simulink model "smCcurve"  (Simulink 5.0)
settings: Solver=ode45  StartTime=0.0  StopTime=0  MaxStep=1  RelTol=1e-6
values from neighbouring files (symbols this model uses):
  Ef = parEf(m)    [Ccurverun.m]
  Ra = .95    (= 0.95)    [altwdgs.m]    (also in Ccurverun.m = 0.018)
  Vs = abs(Vas)    [calc0.m]    (also in Ccurverun.m = 1; IMabc2.m = 1; IMabcrun0.m = Vll*sqrt(2/3); IMabcrun1.m = Vll*sqrt(2/3))
  Xd = 1.15    [Ccurverun.m]
  Xq = 0.75    [Ccurverun.m]
undefined symbols (not defined in the file or in its folder): phi
libraries: simulink x2

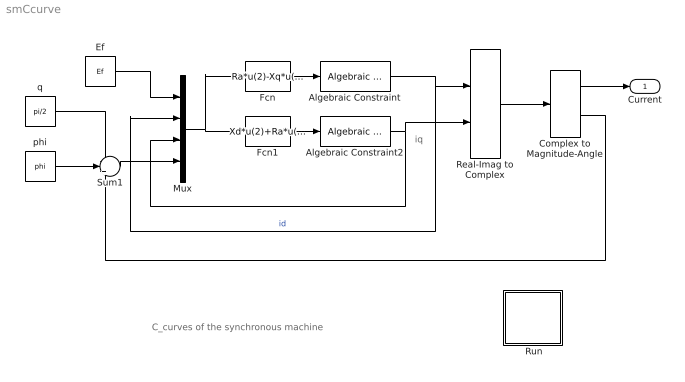
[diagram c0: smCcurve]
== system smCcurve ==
  note: iq
  note: C_curves of the synchronous machine
  " Run" : Subsystem
  Algebraic Constraint : simulink/Math Operations/Algebraic Constraint  z0=.1
  Algebraic Constraint2 : simulink/Math Operations/Algebraic Constraint  z0=0.3
  Complex to Magnitude-Angle : ComplexToMagnitudeAngle
  Ef : Constant  Value=Ef
  Fcn : Fcn  Expr=Ra*u(2)-Xq*u(3)+Vs*sin(u(4))
  Fcn1 : Fcn  Expr=Xd*u(2)+Ra*u(3)-Vs*cos(u(4))+u(1)
  Mux : Mux
  Real-Imag to Complex : RealImagToComplex
  Sum1 : Sum  Inputs=--+
  phi : Constant  Value=phi
  q : Constant  Value=pi/2
  Current : Outport
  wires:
  Mux/1 -> Fcn1/1, Fcn/1
  Ef/1 -> Mux/1
  Fcn/1 -> Algebraic Constraint/1
  Fcn1/1 -> Algebraic Constraint2/1
  Real-Imag to Complex/1 -> Complex to Magnitude-Angle/1
  Algebraic Constraint2/1 -> Real-Imag to Complex/2, Mux/3
  Algebraic Constraint/1 -> Real-Imag to Complex/1, Mux/2  "id"
  q/1 -> Sum1/1
  Complex to Magnitude-Angle/2 -> Sum1/3
  phi/1 -> Sum1/2
  Sum1/1 -> Mux/4
  Complex to Magnitude-Angle/1 -> Current/1

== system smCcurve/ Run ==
  note: Double click the block to enter the machine parameters and run the simulation
  note: This demo illustrates the generation of the compounding C_curvesof a synchronous machine
